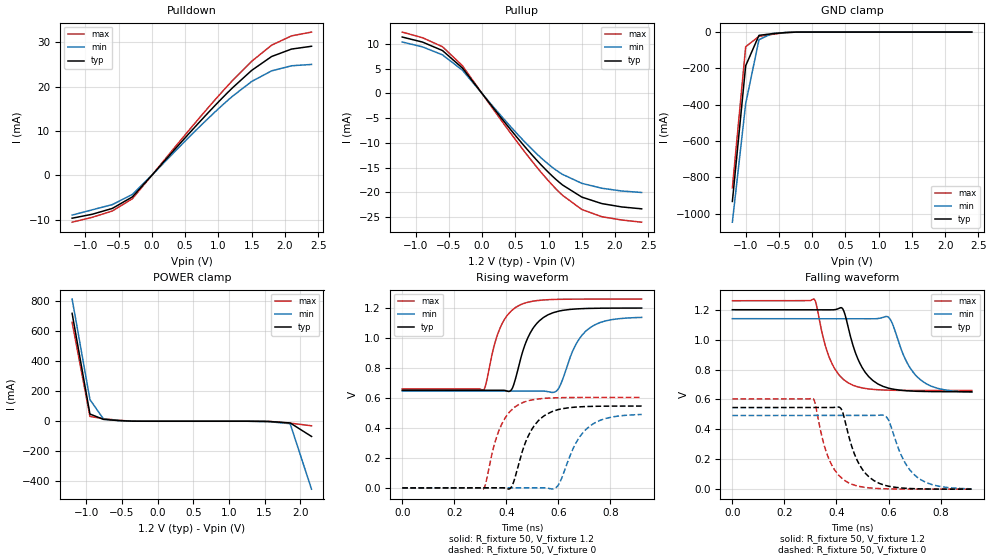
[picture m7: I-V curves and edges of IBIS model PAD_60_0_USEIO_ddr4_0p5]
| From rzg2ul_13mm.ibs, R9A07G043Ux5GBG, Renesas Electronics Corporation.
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|[Package Model]
[Model] PAD_60_0_USEIO_ddr4_0p5
Model_type I/O
Polarity   Non-Inverting
Vinl = 0.5070
Vinh = 0.6930
Vmeas= 0.600
| Capacitance   typ   min   max
C_comp   2.102e-12   2.013e-12   2.214e-12
[Model Spec]
| Subparameter   typ   min   max
Vmeas   0.600   0.570   0.630
Vinh   0.6930   0.6630   0.7230
Vinl   0.5070   0.4770   0.5370
| Variables   typ   min   max
[GND Clamp Reference]   0   0   0
[POWER Clamp Reference]   1.2   1.14   1.26
[Pulldown Reference]   0   0   0
[Pullup Reference]   1.2   1.14   1.26
[Temperature Range]   25   125   -40
[Voltage Range]   1.2   1.14   1.26
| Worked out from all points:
|   slope of the pulldown table from 0 to 0.18 V, typ, clamps not added: 58.8 ohm
|   slope of the pullup table from 0 to 0.18 V, typ, clamps not added: 58 ohm
|   GND clamp passes 1 mA (typ) near -0.30 V on its own axis
|   POWER clamp passes 1 mA (typ) near -0.38 V on its own axis
|   rising waveform, R_fixture 50, V_fixture 1.2: 20-80 % time 73ps typ, 80.7ps min, 66.5ps max; typ from 0.652 V to 1.2 V
|   rising waveform, R_fixture 50, V_fixture 0: 20-80 % time 77.5ps typ, 87.3ps min, 69.9ps max; typ from 0 V to 0.546 V
|   falling waveform, R_fixture 50, V_fixture 1.2: 20-80 % time 75.5ps typ, 84.8ps min, 69.6ps max; typ from 1.2 V to 0.651 V
|   falling waveform, R_fixture 50, V_fixture 0: 20-80 % time 74.1ps typ, 82.6ps min, 67.9ps max; typ from 0.546 V to 0 V
[GND Clamp]
| Voltage   I(typ)   I(min)   I(max)
-1.2V     -932.7mA   -1.047A    -857.4mA
-1V       -185.5mA   -394.3mA   -80.64mA
-800mV    -17.89mA   -41.9mA    -23.65mA
-600mV    -9.04mA    -7.411mA   -12.44mA
-400mV    -2.454mA   -2.378mA   -3.185mA
2.4V      0A         0A         0A
[POWER Clamp]
| Voltage   I(typ)   I(min)   I(max)
-1.2V     719.7mA    815.2mA    660.1mA
-950mV    48.1mA     144.6mA    32.07mA
-760mV    12.41mA    14.91mA    17.11mA
-360mV    527.4uA    791.2uA    575.5uA
1.26V     -115.5nA   -12.89uA   -796.6pA
1.56V     -1.53mA    -2.776mA   -549.4uA
1.86V     -11.39mA   -16.33mA   -12.44mA
2.16V     -101.5mA   -453.2mA   -30.39mA
[Pulldown]
| Voltage   I(typ)   I(min)   I(max)
-1.2V     -9.7mA     -9mA       -10.6mA
-895mV    -8.8mA     -7.8mA     -9.49mA
-595mV    -7.491mA   -6.628mA   -8.07mA
-295mV    -4.902mA   -4.336mA   -5.322mA
855mV     14.25mA    12.95mA    15.4mA
1.21V     19.7mA     17.8mA     21.34mA
1.5V      23.66mA    21.16mA    25.71mA
1.8V      26.79mA    23.55mA    29.35mA
2.1V      28.47mA    24.7mA     31.45mA
2.4V      29.1mA     25mA       32.3mA
[Pullup]
| Voltage   I(typ)   I(min)   I(max)
-1.2V     11.4mA     10.4mA     12.4mA
-895mV    10.38mA    9.41mA     11.26mA
-595mV    8.671mA    7.804mA    9.444mA
-295mV    5.138mA    4.696mA    5.61mA
300mV     -5.138mA   -4.726mA   -5.631mA
650mV     -10.85mA   -9.889mA   -11.94mA
955mV     -15.35mA   -13.8mA    -16.98mA
1.21V     -18.48mA   -16.34mA   -20.57mA
1.5V      -20.93mA   -18.15mA   -23.43mA
1.8V      -22.24mA   -19.14mA   -24.89mA
2.1V      -22.92mA   -19.7mA    -25.56mA
2.4V      -23.3mA    -20mA      -26mA
[Ramp]
dV/dt_r   0.3288/7.302e-11   0.2952/8.066e-11   0.3597/6.654e-11
dV/dt_f   0.3274/7.410e-11   0.2943/8.259e-11   0.3619/6.787e-11
R_load= 50
[Rising Waveform]
R_fixture = 50
V_fixture = 1.2
V_fixture_min = 1.14
V_fixture_max = 1.26
| Time   V(typ)   V(min)   V(max)
0s        651.9mV    645.6mV    660.5mV
312ps     651.9mV    645.6mV    653.2mV
364ps     652.2mV    645.6mV    1.013V
413ps     645mV      645.6mV    1.17V
497ps     1.05V      645.7mV    1.244V
583ps     1.171V     638.2mV    1.257V
608ps     1.182V     688.1mV    1.258V
666ps     1.194V     953.4mV    1.26V
708ps     1.197V     1.05V      1.26V
920ps     1.2V       1.138V     1.26V
[Rising Waveform]
R_fixture = 50
V_fixture = 0
V_fixture_min = 0
V_fixture_max = 0
| Time   V(typ)   V(min)   V(max)
0s        118.2nV    4.925uV    20.55nV
312ps     -1.593uV   4.822uV    -6.708mV
364ps     263.6uV    4.746uV    346.7mV
413ps     -5.676mV   12.71uV    508.5mV
497ps     388.6mV    41.46uV    586.8mV
582ps     513.2mV    -6.19mV    600.9mV
668ps     539.6mV    301.7mV    603.4mV
708ps     543.2mV    393.5mV    603.7mV
780ps     545.5mV    462.7mV    603.9mV
920ps     546.2mV    490mV      603.9mV
[Falling Waveform]
R_fixture = 50
V_fixture = 1.2
V_fixture_min = 1.14
V_fixture_max = 1.26
| Time   V(typ)   V(min)   V(max)
0s        1.2V       1.14V      1.26V
315ps     1.2V       1.14V      1.269V
364ps     1.2V       1.14V      921.3mV
420ps     1.213V     1.14V      745.3mV
497ps     817.9mV    1.14V      677.7mV
596ps     677.3mV    1.153V     662.1mV
670ps     657.9mV    850mV      660.2mV
720ps     653.9mV    735.5mV    659.8mV
788ps     652.1mV    674.5mV    659.7mV
920ps     651.4mV    648.6mV    659.7mV
[Falling Waveform]
R_fixture = 50
V_fixture = 0
V_fixture_min = 0
V_fixture_max = 0
| Time   V(typ)   V(min)   V(max)
0s        545.8mV    492.6mV    603.1mV
310ps     545.8mV    492.6mV    606.4mV
362ps     545.6mV    492.6mV    242.5mV
412ps     547.1mV    492.6mV    87.29mV
488ps     164.2mV    492.5mV    18.1mV
581ps     28.17mV    494mV      2.687mV
602ps     18.98mV    454.9mV    1.67mV
656ps     6.96mV     200.7mV    592.7uV
704ps     2.712mV    88.68mV    189.6uV
920ps     37.71uV    2.199mV    1.697uV
